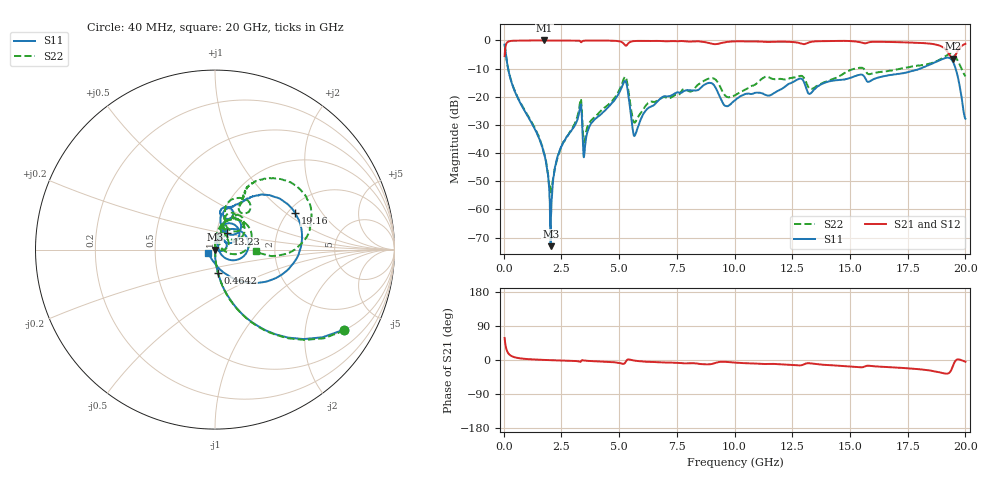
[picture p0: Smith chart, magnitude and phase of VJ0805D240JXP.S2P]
! VJ0805D240JXP
! DATE 10/29/2021  12:21
! CAPACITORS MOUNTED IN SERIES ON 25 MIL THICK MICROSTRIP SUBSTRATE
# GHz  S  MA  R  50.00
!  FREQ  S11M  S11A  S21M  S21A  S12M  S12A  S22M  S22A
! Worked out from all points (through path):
!   1601 points, 40 MHz to 20 GHz, reference 50 ohm
!   highest |S21| = 0.00 dB at 1.762 GHz (marker M1); lowest = -6.4 dB at 19.45 GHz (marker M2)
!   group delay of S21, straight-line fit = 3.82 ps
!   lowest |S11| = -73.1 dB at 2.036 GHz (marker M3), VSWR 1.00, Z = 50 - j0.000414 ohm
!   |S11| at or under -10 dB: 190.5 MHz to 18.05 GHz (17.86 GHz wide, 196 % of centre); 19.58 GHz to end of sweep
!   |S22| runs from -54.0 to -1.4 dB; largest |S21 - S12| = 0.008
!   S11 on the Smith chart (normalised r, x): 40 MHz: 1.02, -3.20; 464.1 MHz: 1.00, -0.26; 13.23 GHz: 1.12, +0.21; 19.16 GHz: 2.19, +1.16; 20 GHz: 0.93, -0.03
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0.04  0.8455 -31.9  0.5273 58.1  0.5275 58.0  0.8504 -32.0
0.202175  0.2995 -72.6  0.9534 17.5  0.9536 17.4  0.3032 -72.7
0.46415  0.1296 -83.0  0.9917 7.4  0.9915 7.4  0.132 -82.9
1.76155  0.009278 -91.3  0.9997 0.2  0.9988 0.1  0.009703 -79.4
2.036  0.0002218 -178.9  0.9984 -0.4  0.9986 -0.5  0.002287 -11.0
2.4352  0.01128 91.1  0.9993 -1.2  0.9987 -1.2  0.0113 82.5
3.271025  0.05303 72.5  0.99 -4.0  0.9903 -4.1  0.06289 82.1
3.370825  0.05808 2.7  0.9349 -1.5  0.935 -1.6  0.07282 12.2
3.533  0.01389 84.9  0.9928 -1.8  0.9939 -1.9  0.01915 79.7
5.242075  0.1893 21.6  0.8338 -8.6  0.8334 -8.7  0.2241 40.8
5.6787  0.02041 19.4  0.9761 -1.7  0.9764 -1.8  0.03472 32.9
6.70165  0.08554 73.3  0.98 -6.0  0.98 -6.1  0.08767 71.6
8.9721  0.1761 44.8  0.8837 -11.0  0.884 -11.1  0.2143 49.5
10.02  0.08643 66.6  0.962 -6.8  0.9628 -7.0  0.1063 60.6
11.3673  0.1069 60.1  0.9422 -10.5  0.9419 -10.6  0.2275 63.3
12.82687  0.2105 54.8  0.8952 -14.3  0.8957 -14.5  0.2337 54.2
13.22607  0.1126 53.2  0.9214 -8.5  0.921 -8.6  0.1425 45.9
13.35083  0.1205 68.3  0.9486 -9.3  0.9488 -9.5  0.1385 58.0
16.68165  0.2399 73.2  0.9397 -18.9  0.9404 -19.1  0.2879 60.9
19.16418  0.4904 24.3  0.6791 -36.1  0.6794 -36.3  0.5333 47.6
19.4511  0.4263 -14.3  0.4775 -17.1  0.4774 -17.4  0.5773 21.6
20  0.04064 -155.4  0.8715 -4.6  0.8707 -5.0  0.2295 -2.0
